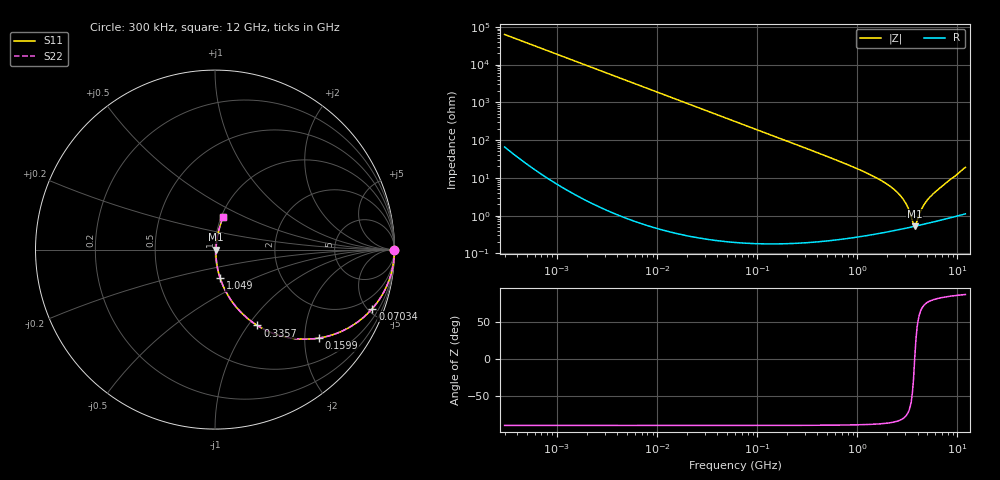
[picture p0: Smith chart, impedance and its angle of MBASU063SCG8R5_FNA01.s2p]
! MBASU063SCG8R5_FNA01  S-PARAMETER MODEL  ( General Type )
! Model Generated by TAIYO YUDEN Corporation (http://www.ty-top.com)
! Version 1.0
! TAIYO YUDEN Control No. 130801
! Copyright(c) 2013 TAIYO YUDEN CO.,LTD. All Rights Reserved.
! Product Description (link to TY-COMPAS)
! https://ds.yuden.co.jp/TYCOMPAS/or/detail?pn=MBASU063SCG8R5DFNA01&u=M
! Products Name : Multilayer Ceramic Capacitors
! Characteristics :
!  Capacitance : 8.5 pF , Rated Voltage : 50V , TCC : CG / C0G
!  Case Size : 0.6 x 0.3 / 0.024 x 0.012 [mm/inch] , Thickness : 0.3 / 0.012 [mm/inch]
!  (Conditions: Temperature = 25 degC , DC Bias Current/Voltage = 0A / 0V)
! External Node Assignments :
!  1  o---| |---o  2
! GND o---------o GND
! Frequency Range : 0.3MHz  -  12000MHz  [ 401 STEP ]
# MHz S RI R 50
! Freq[MHz].  S11 Real  S11 Imag  S21 Real  S21 Imag  S12 Real  S12 Imag  S22 Real  S22 Imag
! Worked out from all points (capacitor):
!   401 points, 300 kHz to 12 GHz, reference 50 ohm
!   read as one part in series: C = 8.48 pF near 316.3 kHz
!   lowest |Z| = 523 mohm at 3.741 GHz (marker M1)
!   series resonance near 3.738 GHz, so ESL is about 210 pH
!   S11 on the Smith chart (normalised r, x): 300 kHz: open; 70.34 MHz: 1.00, -5.33; 159.9 MHz: 1.00, -2.34; 335.7 MHz: 1.00, -1.11; 1.049 GHz: 1.01, -0.33; 12 GHz: 1.02, +0.38
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0.3  1 -0.0016  4.23e-06 0.0016  4.23e-06 0.0016  1 -0.0016
1.769972  0.9999 -0.00943  9.15e-05 0.00943  9.15e-05 0.00943  0.9999 -0.00943
10.44266  0.9969 -0.0555  0.0031 0.0555  0.0031 0.0555  0.9969 -0.0555
27.10171  0.9795 -0.1414  0.0205 0.1414  0.0205 0.1414  0.9795 -0.1414
60  0.9071 -0.29  0.0929 0.29  0.0929 0.29  0.9071 -0.29
70.33673  0.8766 -0.3286  0.1234 0.3286  0.1234 0.3286  0.8766 -0.3286
104.6549  0.7623 -0.4252  0.2377 0.4252  0.2377 0.4252  0.7623 -0.4252
159.8975  0.5784 -0.4931  0.4216 0.4931  0.4216 0.4931  0.5784 -0.4931
335.7268  0.236 -0.4228  0.764 0.4228  0.764 0.4228  0.236 -0.4228
353.9943  0.2172 -0.4105  0.7828 0.4105  0.7828 0.4105  0.2172 -0.4105
570.2811  0.0953 -0.2902  0.9047 0.2902  0.9047 0.2902  0.0953 -0.2902
1048.836  0.029 -0.1596  0.971 0.1596  0.971 0.1596  0.029 -0.1596
2088.533  0.00754 -0.0611  0.9925 0.0611  0.9925 0.0611  0.00754 -0.0611
2514.07  0.00581 -0.0405  0.9942 0.0405  0.9942 0.0405  0.00581 -0.0405
2870.14  0.00518 -0.0266  0.9948 0.0266  0.9948 0.0266  0.00518 -0.0266
3190.978  0.005 -0.0158  0.995 0.0158  0.995 0.0158  0.005 -0.0158
3547.679  0.00507 -0.00522  0.9949 0.00522  0.9949 0.00522  0.00507 -0.00522
3740.715  0.0052 8.36e-05  0.9948 -8.36e-05  0.9948 -8.36e-05  0.0052 8.36e-05
3944.255  0.00539 0.00477  0.9946 -0.00477  0.9946 -0.00477  0.00539 0.00477
4623.766  0.00623 0.0181  0.9938 -0.0181  0.9938 -0.0181  0.00623 0.0181
5278.635  0.00729 0.0296  0.9927 -0.0296  0.9927 -0.0296  0.00729 0.0296
12000  0.0449 0.1798  0.9551 -0.1798  0.9551 -0.1798  0.0449 0.1798
